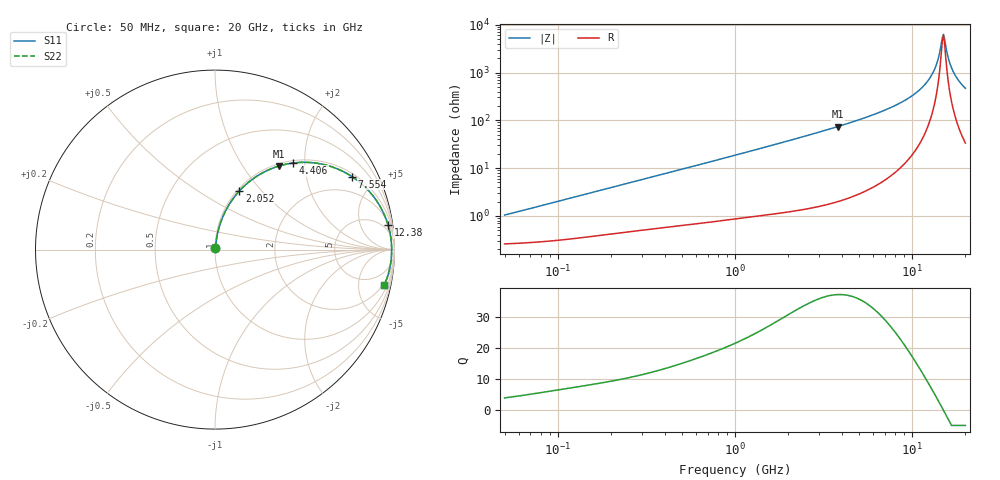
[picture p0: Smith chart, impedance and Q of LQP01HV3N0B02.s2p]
!Murata Part Number: LQP01HV3N0B02
!These Parameters are Measured in Series Mode Connection
!  o--[Z]--o
!Port1  Port2
!  o-------o
!Freq. Start=50[MHz] Stop=20[GHz], 401[Steps]
# Hz S RI R 50
!Freq.(Hz) S11(Real) S11(Imag) S21(Real) S21(Imag) S12(Real) S12(Imag) S22(Real) S22(Imag)
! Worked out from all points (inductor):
!   401 points, 50 MHz to 20 GHz, reference 50 ohm
!   read as one part in series: L = 3.2 nH near 51.52 MHz
!   highest Q = 37.2 at 3.793 GHz (marker M1), where L = 3.09 nH
!   self-resonance near 14.82 GHz
!   S11 on the Smith chart (normalised r, x): 50 MHz: 1.01, +0.02; 2.052 GHz: 1.02, +0.76; 4.406 GHz: 1.05, +1.75; 7.554 GHz: 1.14, +3.67; 12.38 GHz: 3, +14; 20 GHz: 1.67, -9.33
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5e7  0.00269 0.01  0.9973 -0.01  0.9973 -0.01  0.00269 0.01
1.364002e8  0.00421 0.0267  0.9958 -0.0267  0.9958 -0.0267  0.00421 0.0267
3.721004e8  0.0104 0.0695  0.9896 -0.0695  0.9896 -0.0695  0.0104 0.0695
1e9  0.041 0.1764  0.959 -0.1764  0.959 -0.1764  0.041 0.1764
2.05233e9  0.1352 0.3262  0.8648 -0.3262  0.8648 -0.3262  0.1352 0.3262
2.728004e9  0.2156 0.3972  0.7844 -0.3972  0.7844 -0.3972  0.2156 0.3972
3.792786e9  0.3555 0.4654  0.6445 -0.4654  0.6445 -0.4654  0.3555 0.4654
4.405649e9  0.436 0.4825  0.564 -0.4825  0.564 -0.4825  0.436 0.4825
5.769027e9  0.5988 0.4755  0.4012 -0.4755  0.4012 -0.4755  0.5988 0.4755
7.442007e9  0.7543 0.4126  0.2457 -0.4126  0.2457 -0.4126  0.7543 0.4126
7.554318e9  0.7629 0.4071  0.2371 -0.4071  0.2371 -0.4071  0.7629 0.4071
1.019291e10  0.9082 0.26  0.0918 -0.26  0.0918 -0.26  0.9082 0.26
1.238412e10  0.9648 0.135  0.0352 -0.135  0.0352 -0.135  0.9648 0.135
1.354865e10  0.9786 0.0727  0.0214 -0.0727  0.0214 -0.0727  0.9786 0.0727
1.396067e10  0.9814 0.0516  0.0186 -0.0516  0.0186 -0.0516  0.9814 0.0516
1.460232e10  0.9838 0.0198  0.0162 -0.0198  0.0162 -0.0198  0.9838 0.0198
1.504638e10  0.9843 -0.0015  0.0157 0.0015  0.0157 0.0015  0.9843 -0.0015
1.527346e10  0.9842 -0.0122  0.0158 0.0122  0.0158 0.0122  0.9842 -0.0122
1.621653e10  0.9815 -0.0547  0.0185 0.0547  0.0185 0.0547  0.9815 -0.0547
1.696185e10  0.977 -0.0863  0.023 0.0863  0.023 0.0863  0.977 -0.0863
1.828096e10  0.965 -0.1382  0.035 0.1382  0.035 0.1382  0.965 -0.1382
2e10  0.9433 -0.1982  0.0567 0.1982  0.0567 0.1982  0.9433 -0.1982
